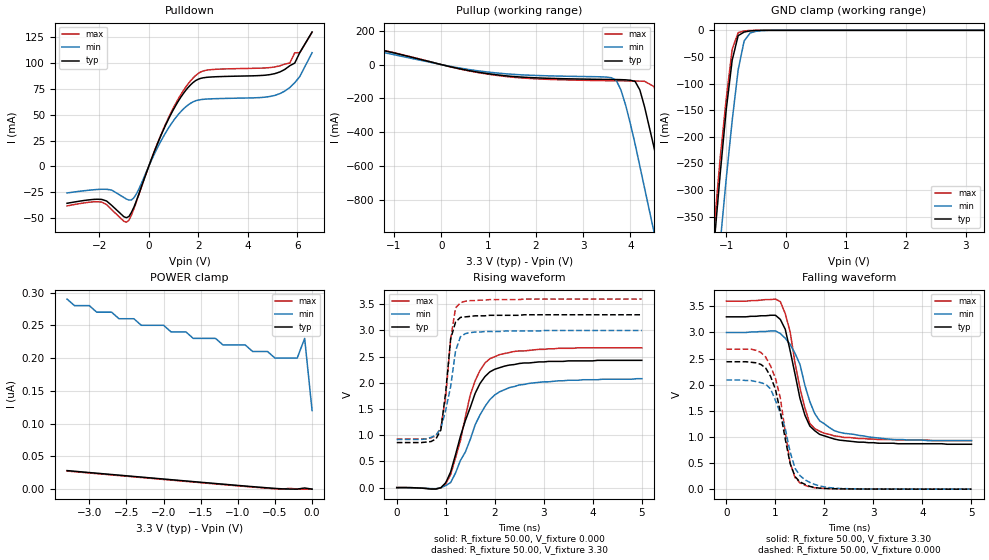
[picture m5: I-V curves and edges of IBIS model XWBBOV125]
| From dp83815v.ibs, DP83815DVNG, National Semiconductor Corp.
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|   Model XWBBOV125
[Model]   XWBBOV125
Model_type   I/O
Polarity   Non-Inverting
Enable   Active-High
Vinl =   0.80V
Vinh =   2.00V
Vmeas =   1.50V
Cref =  20.00pF
Rref = 100.00k
C_comp   5.00pF   5.00pF   5.00pF
[Temperature Range]   25.00   0.14k   0.000
[Voltage Range]   3.30V   3.00V   3.60V
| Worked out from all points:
|   slope of the pulldown table from 0 to 0.495 V, typ, clamps not added: 16.5 ohm
|   slope of the pullup table from 0 to 0.495 V, typ, clamps not added: 16.1 ohm
|   GND clamp passes 1 mA (typ) near -0.58 V on its own axis
|   rising waveform, R_fixture 50.00, V_fixture 0.000: 20-80 % time 519ps typ, 631ps min, 459ps max; typ from 0 V to 2.43 V
|   rising waveform, R_fixture 50.00, V_fixture 3.30: 20-80 % time 163ps typ, 237ps min, 185ps max; typ from 0.86 V to 3.3 V
|   falling waveform, R_fixture 50.00, V_fixture 3.30: 20-80 % time 374ps typ, 469ps min, 348ps max; typ from 3.3 V to 0.86 V
|   falling waveform, R_fixture 50.00, V_fixture 0.000: 20-80 % time 318ps typ, 383ps min, 304ps max; typ from 2.44 V to 0 V
[Pulldown]
| voltage   I(typ)   I(min)   I(max)
-3.3V     -35.71mA   -25.71mA   -38.23mA
-1.9V     -31.94mA   -22.12mA   -34.55mA
-900mV    -49.65mA   -31.63mA   -54mA
-500mV    -33.54mA   -26.73mA   -34.28mA
800mV     45.8mA     37.13mA    47.07mA
1.8V      81.34mA    62.58mA    85.74mA
2.4V      86.32mA    65.25mA    93.37mA
5.3V      91.42mA    70.44mA    97.34mA
5.7V      97.45mA    76.39mA    100mA
5.9V      100mA      81.01mA    110mA
6.1V      110mA      86.87mA    110mA
6.6V      130mA      110mA      130mA
[Pullup]
| voltage   I(typ)   I(min)   I(max)
-3.3V     200mA      170mA      210mA
900mV     -50.23mA   -41.2mA    -52.73mA
3.6V      -88.17mA   -77.78mA   -95.51mA
3.7V      -88.52mA   -93mA      -95.87mA
3.9V      -90.24mA   -240mA     -96.54mA
4.1V      -99.64mA   -470mA     -97.17mA
4.3V      -250mA     -730mA     -98.85mA
4.5V      -490mA     -990mA     -130mA
4.9V      -1.02A     -1.53A     -600mA
5.1V      -1.3A      -1.8A      -870mA
5.3V      -1.57A     -2.07A     -1.14A
6.6V      -3.39A     -3.87A     -2.95A
[GND_clamp]
| voltage   I(typ)   I(min)   I(max)
-3.3V     -3.28A     -3.36A     -3.26A
-1.2V     -400mA     -520mA     -370mA
-1.1V     -270mA     -400mA     -240mA
-1V       -150mA     -280mA     -130mA
-900mV    -56.24mA   -170mA     -35.64mA
-800mV    -9.97mA    -74.34mA   -4.49mA
-700mV    -3.19mA    -19.87mA   -1.15mA
-600mV    -1.14mA    -5mA       -210uA
-500mV    -210uA     -1.78mA    -18.22uA
-200mV    -44.3nA    -11.19uA   -980pA
3.3V      93.97pA    200nA      36.14pA
[POWER_clamp]
| voltage   I(typ)   I(min)   I(max)
-3.3V     28.36nA    290nA      27.7nA
-2.7V     22.4nA     270nA      21.75nA
-2.6V     21.41nA    260nA      20.76nA
-2.4V     19.44nA    260nA      18.78nA
-2.3V     18.45nA    250nA      17.79nA
-2V       15.49nA    250nA      14.84nA
-1.6V     11.56nA    230nA      10.91nA
-900mV    4.8nA      220nA      4.15nA
-500mV    1.21nA     200nA      640pA
-200mV    120pA      200nA      190pA
-100mV    1.86nA     230nA      45.35pA
0V        93.97pA    120nA      39.6pA
[Ramp]
| variable   typ   min   max
dV/dt_r   1.92/0.26n   1.74/0.34n   2.10/0.26n
dV/dt_f   1.92/0.27n   1.73/0.37n   2.10/0.26n
R_load = 0.50k
[Rising Waveform]
R_fixture = 50.00
V_fixture = 0.000
V_fixture_min = 0.000
V_fixture_max = 0.000
| time   V(typ)   V(min)   V(max)
0s        130uV      120uV      150uV
800ps     -25.54mV   -20.43mV   -29.49mV
1ns       93.68mV    39.31mV    72.43mV
1.2ns     630mV      280mV      570mV
1.5ns     1.53V      920mV      1.77V
1.6ns     1.8V       1.2V       2.04V
1.9ns     2.21V      1.68V      2.46V
2.3ns     2.34V      1.91V      2.58V
2.7ns     2.38V      1.99V      2.62V
5ns       2.43V      2.08V      2.67V
[Rising Waveform]
R_fixture = 50.00
V_fixture = 3.30
V_fixture_min = 3.00
V_fixture_max = 3.60
| time   V(typ)   V(min)   V(max)
0s        860mV      920mV      930mV
700ps     880mV      960mV      950mV
800ps     930mV      1V         990mV
900ps     1.1V       1.13V      1.15V
1ns       1.83V      1.48V      1.74V
1.1ns     2.84V      1.93V      2.84V
1.2ns     3.16V      2.61V      3.43V
1.3ns     3.25V      2.88V      3.53V
1.8ns     3.28V      2.98V      3.58V
5ns       3.3V       3V         3.6V
[Falling Waveform]
R_fixture = 50.00
V_fixture = 3.30
V_fixture_min = 3.00
V_fixture_max = 3.60
| time   V(typ)   V(min)   V(max)
0s        3.3V       3V         3.6V
1.1ns     3.25V      2.98V      3.59V
1.2ns     3.06V      2.89V      3.36V
1.3ns     2.65V      2.77V      3.01V
1.5ns     1.74V      2.39V      1.94V
1.6ns     1.42V      1.99V      1.56V
1.7ns     1.21V      1.68V      1.26V
1.8ns     1.12V      1.45V      1.16V
2.4ns     930mV      1.07V      990mV
5ns       860mV      930mV      930mV
[Falling Waveform]
R_fixture = 50.00
V_fixture = 0.000
V_fixture_min = 0.000
V_fixture_max = 0.000
| time   V(typ)   V(min)   V(max)
0s        2.44V      2.09V      2.68V
600ps     2.42V      2.06V      2.66V
900ps     2.16V      1.92V      2.36V
1ns       1.91V      1.7V       2.12V
1.1ns     1.48V      1.45V      1.74V
1.3ns     490mV      710mV      500mV
1.4ns     240mV      400mV      220mV
1.5ns     140mV      260mV      120mV
2.2ns     8.63mV     21.49mV    9.11mV
5ns       250uV      370uV      270uV
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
